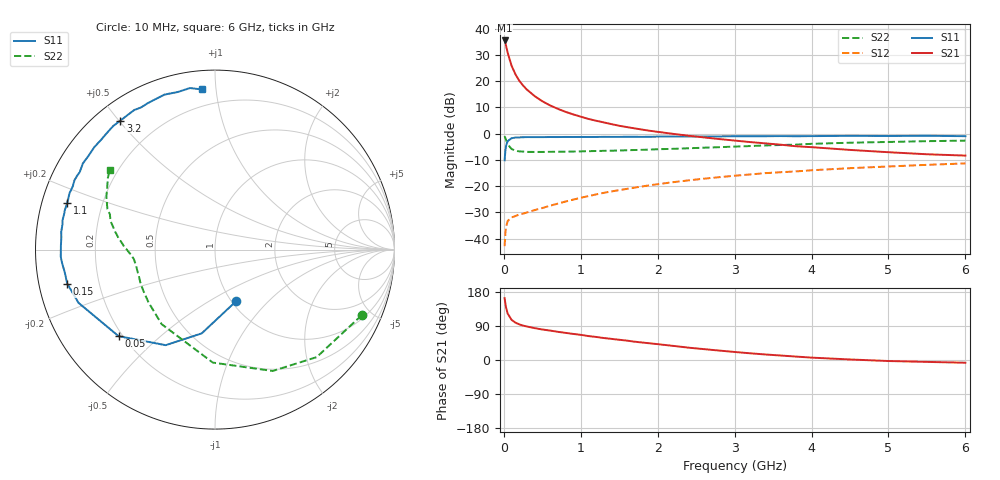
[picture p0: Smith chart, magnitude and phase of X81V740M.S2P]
! SIEMENS Small Signal Semiconductors
! BFP136W
! Si NPN RF Bipolar Junction Transistor in SOT343
! VCE = 1.75 V  IC = 40 mA
! Common Emitter S-Parameters:  September  1994
# GHz  S  MA  R  50
!  f  S11  S21  S12  S22
! GHz  MAG  ANG  MAG  ANG  MAG  ANG  MAG  ANG
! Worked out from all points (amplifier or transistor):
!   40 points, 10 MHz to 6 GHz, reference 50 ohm
!   highest |S21| = 35.5 dB at 10 MHz (marker M1)
!   |S21| within 3 dB of that: start of sweep to 36.59 MHz
!   unconditionally stable (mu >= 1): 649.1 MHz to 2.86 GHz
!   at 200 MHz: K = 0.51, MSG = 25.5 dB, |S12| = -30.8 dB
!   at 1.5 GHz: K = 1.14, MAG = 10.0 dB, |S12| = -21.5 dB
!   at 6 GHz: K = 0.97, MSG = 1.5 dB, |S12| = -11.3 dB
!   S11 on the Smith chart (normalised r, x): 10 MHz: 1.04, -0.67; 50 MHz: 0.18, -0.37; 150 MHz: 0.09, -0.11; 1.1 GHz: 0.07, +0.15; 3.2 GHz: 0.07, +0.50; 6 GHz: 0.10, +0.92
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0.01  0.3113 -68.1  59.51 163.3  0.0072 72.2  0.8955 -24.1
0.02  0.4725 -99.0  52.96 148.6  0.0129 60.2  0.8245 -46.6
0.03  0.5993 -117.3  46.42 137.3  0.017 51.4  0.7486 -64.6
0.05  0.7219 -138.1  34.59 122.4  0.0217 39.7  0.6297 -91.1
0.1  0.8162 -158.7  19.75 106.1  0.0254 30.2  0.5108 -125.6
0.15  0.8449 -167.0  13.55 98.6  0.027 30.0  0.473 -141.5
0.2  0.8467 -171.5  10.2 94.1  0.0289 31.1  0.4603 -150.4
0.25  0.8554 -175.0  8.244 90.8  0.03 32.9  0.4548 -156.1
0.3  0.8602 -177.3  6.895 88.4  0.0316 35.1  0.4499 -159.9
0.4  0.8589 178.6  5.194 84.1  0.035 39.9  0.4484 -164.8
0.5  0.8586 175.5  4.141 80.5  0.0383 43.2  0.4486 -168.0
0.6  0.8624 173.4  3.456 77.7  0.0424 46.6  0.4501 -169.9
0.7  0.8613 170.7  2.977 74.4  0.0464 49.2  0.4522 -171.3
0.9  0.8637 166.9  2.329 68.9  0.0553 52.4  0.4563 -173.7
1.1  0.8635 162.5  1.906 63.1  0.0647 54.4  0.4632 -175.2
1.5  0.8672 156.0  1.413 53.4  0.0841 56.1  0.4777 -177.9
1.8  0.8685 150.2  1.193 46.1  0.0989 55.4  0.4918 179.9
2.2  0.8774 143.5  0.991 37.3  0.1189 53.6  0.5138 176.9
3.2  0.8915 126.3  0.692 17.7  0.1671 45.8  0.5803 167.6
4.5  0.9083 108.1  0.49 1.4  0.2199 34.0  0.6722 154.2
5.5  0.9109 98.8  0.405 -5.0  0.2546 25.9  0.719 146.1
6  0.8949 94.6  0.382 -7.2  0.2713 21.5  0.7361 142.7
